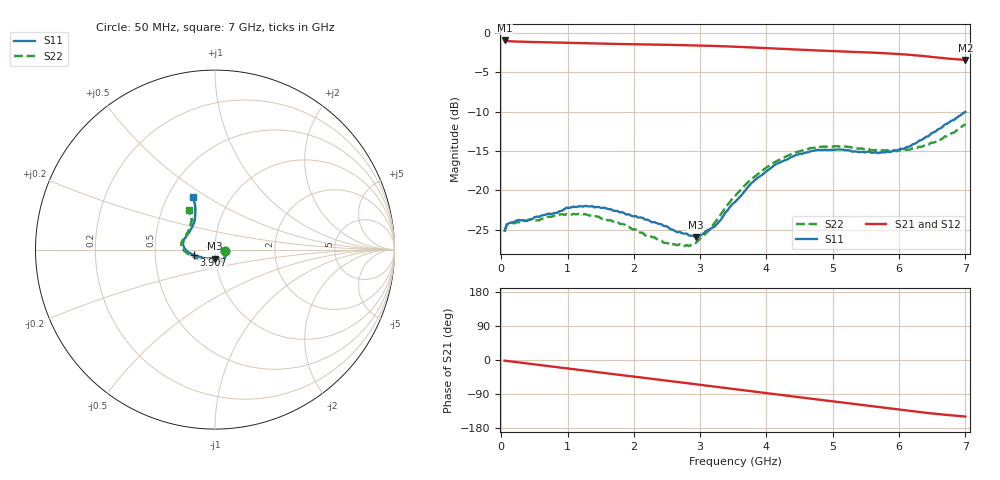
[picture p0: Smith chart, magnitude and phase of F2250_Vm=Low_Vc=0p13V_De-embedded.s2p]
! Integrated Device Technology
! Corporate Headquarters
! 6024 Silver Creek Valley Road
! San Jose, CA 95138  USA
! Phone:  1-408-284-8200
! Toll Free:  1-800-223-1366
! Webpage:  http://www.idt.com/
! Timing and RF Division
! 515 Groton Road, Suite 102
! Westford, MA 01886-6024
! Device:  F2250
! Description: Voltage Variable RF Attenuator
! Frequency:  50.0 -  6000.00 MHz
! Package:  3x3 mm Thin QFN Plastic Package: 16 pin
! Ports:  2 RF, 3 DC
!  Pin  1  = GND
!  Pin  2  = NC
!  Pin  3  = RF1  = Port 1
!  Pin  4  = NC
!  Pin  5  = GND
!  Pin  6  = GND
!  Pin  7  = GND
!  Pin  8  = GND
!  Pin  9  = NC
!  Pin 10  = RF2  = Port 2
!  Pin 11  = NC
!  Pin 12  = GND
!  Pin 13  = GND
!  Pin 14  = VCNTRL
!  Pin 15  = VDD
!  Pin 16  = VMODE
! Vcntrl:  0.130 Volts
! Vmode:  +0.000 Volts
! Vdd:  +3.30  Volts
! Current:  1.108 mA
! Data:  The device was measured on a the F2250 evaluation board which has
!  individual transmission lines to the RF pins.  Data was collected
!  using a calibrated network analyzer.  The evaluation board was
!  de-embedded using a TRL calibration technique.
!  The reference plane is the edge of the package pin.
! Misc:  SN 10
!  Action Tracker AT0258
! Date Measured:  2014-11-26
! Date:  2015-10-15  MJV
! Note:
!  Integrated Device Technology supplies this data as a sample of measured
!  data at the package pin for this product.  Your particular data for this
!  product may vary.
!  Data was taken at 25 degrees C.
!  Integrated Device Technology reserves the right to change this data at anytime.
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# GHz S dB R 50
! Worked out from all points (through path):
!   201 points, 50 MHz to 7 GHz, reference 50 ohm
!   highest |S21| = -0.93 dB at 50 MHz (marker M1); lowest = -3.4 dB at 7 GHz (marker M2)
!   group delay of S21, straight-line fit = 60 ps
!   lowest |S11| = -26.0 dB at 2.934 GHz (marker M3), VSWR 1.11, Z = 49.5 - j4.99 ohm
!   |S11| at or under -10 dB: start of sweep to end of sweep
!   |S22| runs from -27.1 to -11.6 dB; largest |S21 - S12| = 0.00032
!   S11 on the Smith chart (normalised r, x): 50 MHz: 1.12, -0.02; 3.907 GHz: 0.79, -0.05; 7 GHz: 0.67, +0.43
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0.05  -25.12 -9.7  -0.93 -1.8  -0.93 -1.8  -25.23 -10.1
0.08475  -24.29 -9.7  -0.99 -2.5  -0.99 -2.5  -24.34 -9.4
0.15425  -24.07 -11.9  -1.04 -4.0  -1.04 -4.0  -24.10 -11.1
0.57125  -23.35 -30.1  -1.14 -13.1  -1.14 -13.1  -23.82 -30.4
0.884  -22.62 -45.9  -1.20 -19.9  -1.20 -19.9  -23.05 -46.9
1.2315  -22.06 -56.1  -1.28 -27.4  -1.28 -27.4  -23.05 -59.7
1.75275  -22.62 -62.8  -1.37 -38.4  -1.37 -38.4  -23.95 -66.7
2.37825  -24.25 -63.6  -1.46 -51.8  -1.46 -51.8  -26.30 -67.8
2.552  -24.94 -67.8  -1.49 -55.6  -1.49 -55.6  -26.95 -73.3
2.83  -25.72 -83.3  -1.54 -61.7  -1.54 -61.7  -27.07 -92.6
2.93425  -25.97 -92.4  -1.56 -64.0  -1.56 -64.0  -26.69 -101.5
3.21225  -24.62 -122.1  -1.63 -70.1  -1.63 -70.1  -24.17 -127.6
3.525  -21.47 -148.3  -1.72 -77.0  -1.72 -77.0  -20.72 -146.4
3.76825  -19.10 -161.3  -1.81 -82.4  -1.81 -82.4  -18.56 -156.7
3.90725  -18.17 -165.6  -1.87 -85.4  -1.87 -85.4  -17.67 -162.9
4.1505  -16.61 -173.7  -1.97 -90.7  -1.97 -90.8  -16.27 -171.4
4.7065  -14.96 172.2  -2.18 -102.8  -2.18 -102.8  -14.60 175.7
5.15825  -14.82 161.5  -2.33 -112.5  -2.33 -112.5  -14.36 166.5
5.85325  -15.09 138.4  -2.58 -127.4  -2.58 -127.4  -15.00 151.5
6.166  -14.40 127.6  -2.75 -134.2  -2.76 -134.2  -14.81 142.7
6.444  -13.10 119.3  -2.96 -140.0  -2.96 -140.0  -14.19 133.3
7  -10.01 113.0  -3.41 -149.3  -3.41 -149.3  -11.59 123.9
